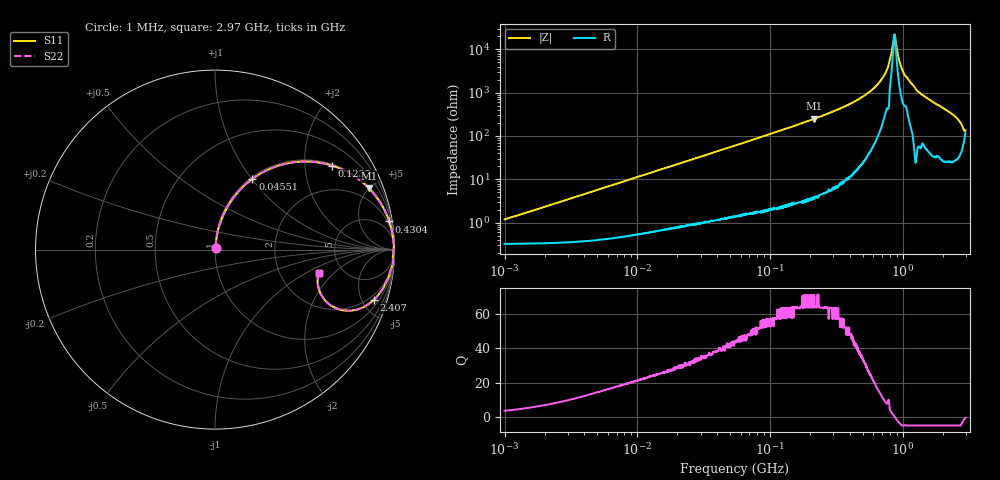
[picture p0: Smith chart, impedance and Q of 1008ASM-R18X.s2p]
!s-Parameter Generated by FASTRON Sdn. Bhd.
!FASTRON P/N : 1008ASM-R18X
!Keysight Technologies: E4991B_MY54100416_A.01.15
!Date: Mon Nov 20 16:15:23 2023
!Version  :Rev00  Wed Nov 22 15:13:17 2023
!Data & Calibration Information:
!Freq  S11  S21  S12  S22
!PortZ  Port1:50+j0  Port2:50+j0
!When reading reference impedance value at option line is always used.
! Remarks : This data is being provided solely for informational purposes.
# Hz S dB R 50
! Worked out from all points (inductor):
!   1599 points, 1 MHz to 2.97 GHz, reference 50 ohm
!   read as one part in series: L = 183 nH near 1.036 MHz
!   highest Q = 63.9 at 215.8 MHz (marker M1), where L = 184 nH
!   self-resonance near 867.3 MHz
!   S11 on the Smith chart (normalised r, x): 1 MHz: 1.01, +0.02; 45.51 MHz: 1.03, +1.01; 123.2 MHz: 1.05, +2.75; 430.4 MHz: 1, +12; 2.407 GHz: 1.51, -6.09; 2.97 GHz: 3.34, -1.31
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1000000  -38.50 73.6  -0.03 -0.7  -0.03 -0.7  -38.50 73.6
3804036  -27.30 82.7  -0.04 -2.5  -0.04 -2.5  -27.30 82.7
1.439846e7  -16.00 78.6  -0.17 -9.1  -0.17 -9.1  -16.00 78.6
4.551475e7  -7.03 62.1  -1.07 -26.4  -1.07 -26.4  -7.03 62.1
5.477226e7  -5.80 57.9  -1.44 -30.8  -1.44 -30.8  -5.80 57.9
1.232024e8  -1.92 35.7  -4.67 -53.3  -4.67 -53.3  -1.92 35.7
2.073156e8  -0.75 22.6  -8.32 -66.6  -8.32 -66.6  -0.75 22.6
2.157832e8  -0.69 21.7  -8.65 -67.5  -8.65 -67.5  -0.69 21.7
4.304467e8  -0.14 9.2  -16.00 -79.5  -16.00 -79.5  -0.14 9.2
6.423554e8  -0.05 3.8  -23.70 -82.8  -23.70 -82.8  -0.05 3.8
7.316083e8  -0.04 2.1  -28.40 -81.6  -28.40 -81.6  -0.04 2.1
7.846996e8  -0.02 1.2  -33.20 -83.1  -33.20 -83.1  -0.02 1.2
8.501091e8  -0.04 0.3  -43.80 -46.4  -43.80 -46.4  -0.04 0.3
8.71647e8  -0.04 -0.0  -46.70 8.1  -46.70 8.1  -0.04 -0.0
8.892696e8  -0.04 -0.3  -43.40 46.0  -43.40 46.0  -0.04 -0.3
9.443041e8  -0.05 -1.0  -34.60 73.2  -34.60 73.2  -0.05 -1.0
9.878038e8  -0.05 -1.6  -30.90 77.2  -30.90 77.2  -0.05 -1.6
1.142072e9  -0.06 -3.2  -24.90 81.1  -24.90 81.1  -0.06 -3.2
1.374365e9  -0.10 -6.1  -19.50 80.7  -19.50 80.7  -0.10 -6.1
2.407135e9  -0.65 -17.6  -10.40 67.6  -10.40 67.6  -0.65 -17.6
2.769173e9  -1.86 -24.9  -7.27 51.8  -7.27 51.8  -1.86 -24.9
2.970126e9  -4.56 -12.5  -7.10 16.8  -7.10 16.8  -4.56 -12.5
